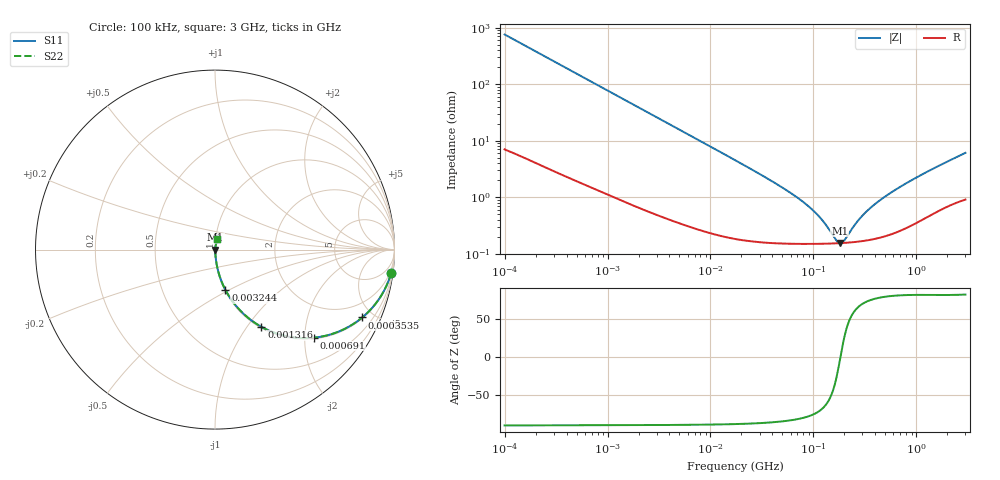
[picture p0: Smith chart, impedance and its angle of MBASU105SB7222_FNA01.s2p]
! MBASU105SB7222_FNA01  S-PARAMETER MODEL  ( Standard Model )
! Model Generated by TAIYO YUDEN Corporation (http://www.ty-top.com)
! Version 1.0
! TAIYO YUDEN Control No. 220601
! Copyright(c) 2013 TAIYO YUDEN CO.,LTD. All Rights Reserved.
! Product Description (link to TY-COMPAS)
! https://ds.yuden.co.jp/TYCOMPAS/or/detail?pn=MBASU105SB7222KFNA01&u=M
! Products Name : Multilayer Ceramic Capacitors
! Characteristics :
!  Capacitance : 2200 [pF] , Rated Voltage : 50 [V] , TCC : X7R
!  Case Size : 1.0 x 0.5 / 0.039 x 0.02 [mm/inch] , Thickness : 0.5 / 0.02 [mm/inch]
!  (Conditions: Temperature = 25 [degC] , DC Bias Voltage = 0 [V])
! External Node Assignments :
!  1  o---| |---o  2
! GND o---------o GND
! Frequency Range : 100kHz  -  3GHz  [ 401 STEP ]
# MHZ S RI R 50
! Freq[MHz].  S11 Real  S11 Imag  S21 Real  S21 Imag  S12 Real  S12 Imag  S22 Real  S22 Imag
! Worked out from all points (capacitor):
!   401 points, 100 kHz to 3 GHz, reference 50 ohm
!   read as one part in series: C = 2.1 nF near 105.3 kHz
!   lowest |Z| = 153 mohm at 180.8 MHz (marker M1)
!   series resonance near 183.4 MHz, so ESL is about 360 pH
!   S11 on the Smith chart (normalised r, x): 100 kHz: 1, -15; 353.5 kHz: 1.05, -4.32; 691 kHz: 1.03, -2.22; 1.316 MHz: 1.02, -1.17; 3.244 MHz: 1.01, -0.48; 3 GHz: 1.02, +0.12
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0.1  0.9817 -0.1295  0.0183 0.1295  0.0183 0.1295  0.9817 -0.1295
0.205778  0.9295 -0.2507  0.0705 0.2507  0.0705 0.2507  0.9295 -0.2507
0.353547  0.8206 -0.3779  0.1794 0.3779  0.1794 0.3779  0.8206 -0.3779
0.562235  0.6482 -0.4712  0.3518 0.4712  0.3518 0.4712  0.6482 -0.4712
0.690972  0.5516 -0.4907  0.4484 0.4907  0.4484 0.4907  0.5516 -0.4907
1.316074  0.259 -0.4305  0.741 0.4305  0.741 0.4305  0.259 -0.4305
1.987766  0.1359 -0.3344  0.8641 0.3344  0.8641 0.3344  0.1359 -0.3344
3.161081  0.0609 -0.2299  0.9391 0.2299  0.9391 0.2299  0.0609 -0.2299
3.243608  0.0582 -0.2248  0.9418 0.2248  0.9418 0.2248  0.0582 -0.2248
7.027689  0.0149 -0.1094  0.9851 0.1094  0.9851 0.1094  0.0149 -0.1094
17.7727  0.00371 -0.0437  0.9963 0.0437  0.9963 0.0437  0.00371 -0.0437
53.83243  0.00168 -0.0134  0.9983 0.0134  0.9983 0.0134  0.00168 -0.0134
97.38194  0.00151 -0.00582  0.9985 0.00582  0.9985 0.00582  0.00151 -0.00582
126.0104  0.0015 -0.0033  0.9985 0.0033  0.9985 0.0033  0.0015 -0.0033
167.3121  0.00152 -0.000788  0.9985 0.000788  0.9985 0.000788  0.00152 -0.000788
180.7614  0.00153 -0.000122  0.9985 0.000122  0.9985 0.000122  0.00153 -0.000122
200.3904  0.00154 0.000765  0.9985 -0.000765  0.9985 -0.000765  0.00154 0.000765
259.3015  0.00162 0.00304  0.9984 -0.00304  0.9984 -0.00304  0.00162 0.00304
318.6746  0.00171 0.00498  0.9983 -0.00498  0.9983 -0.00498  0.00171 0.00498
547.5153  0.00226 0.0112  0.9977 -0.0112  0.9977 -0.0112  0.00226 0.0112
1156.079  0.00461 0.025  0.9954 -0.025  0.9954 -0.025  0.00461 0.025
3000  0.0124 0.0588  0.9876 -0.0588  0.9876 -0.0588  0.0124 0.0588
